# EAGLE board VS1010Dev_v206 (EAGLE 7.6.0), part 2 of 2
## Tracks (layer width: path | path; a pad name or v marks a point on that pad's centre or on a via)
3V3  (via drill 0.5)
  Top 0.2: R7.1 v96.1,27.6
  Top 0.305: C31.1 93.2,25.5 92.35,26.35 90.44,26.35 | C31.1 93.25,25.65 94.95,27.35 R7.1 | C31.1 R8.1 93.25,23.25 93.2,23.2 | CN3.4 90.35,26.35 v90.4,26.3
  Top 0.61: C37.1 29.1,20.8 29.05,20.75 U5.5 | 90.44,26.35 90.44,26.34 v90.4,26.3
  Top 1.016: C37.1 30.45,20.75 v30.5,20.8
  PWR 0.607: v96.1,27.6 96.1,34.72 JP15.7
  PWR 0.61: v30.5,20.8 37.6,20.8 39.4,22.6 40.7,22.6 42.4,20.9 42.4,15.8 43.5,14.7 47.1,14.7 50.8,18.4 50.8,19.3 52.6,21.1 60.6,21.1 61.7,22.2 81.6,22.2 85.7,26.3 v90.4,26.3
4V5  (via drill 0.5, 0.6)
  Top 0.203: U30.5 61.35,44.15 60.5,45 59.7,45 59,45.7 59,45.85 C61.2
  Top 0.25: U7.3 38.1,47.2 38.5,47.6 | 38.75,47.65 C19.1 38.5,47.6 | v39.6,48.5 39.4,48.5 38.5,47.6 | C39.1 34,51.3 34.2,51.1 U7.9 | v29.7,48.5 30.55,47.65 C17.1 30.8,47.6 31.2,47.2 U7.13 | J1.3 v30,41.2
  Top 0.305: 30.5,30.8 v32,30.8 v32,31.9 | v32,31.9 v32,33 | 30.5,30.9 30.8,30.9 31.8,31.9 v32,31.9 | J2.3 v39.2,41.2
  Top 0.406: C39.1 34.15,51.35 34.4,51.6 34.7,51.6 | 34.7,51.6 35.5,51.6 35.6,51.5 v35.6,51.4 v35.6,52.5 | 34.7,51.6 34.7,51.7 35.5,52.5 35.5,52.1 35.3,51.9 35.3,51.4 34.7,51.4
  Top 0.5: U8.6 30.14,31.16 30.5,30.8
  Top 0.6: 30.5,32.7 R21.2 30.5,30.9 C47.2 30.5,30.8
  Top 0.61: C61.2 C59.2 56.25,46.15 v56,45.9
  PWR 0.61: v39.6,48.5 39.6,48.6 39.7,48.5 46.8,48.5 48.2,47.1 48.2,46.1 49.8,44.5 54.6,44.5 v56,45.9
  pour PWR: 29.3,30.2 32.7,30.2 32.7,40.3 39.7,40.3 39.7,53.1 29.3,53.1
14
  Top 0.2: 52,24.2 52.9,23.3 54.4,23.3 56.2,21.5 57.2,21.5 59.3,19.4 59.3,13.1 60.5,11.9 63.3,11.9 64.5,10.7 64.5,2.4 64.9,2 79.6,2 80.3,2.7 80.3,10.6 85.05,15.35 85.05,15.45 R53.2 85.15,15.45 85.1,15.4
  Top 0.203: U6.14 52,24.2
16
  Top 0.2: 52.8,24 53.1,23.7 54.6,23.7 56.4,21.9 57.4,21.9 59.7,19.6 59.7,13.3 60.7,12.3 63.6,12.3 65,10.9 65,2.8 65.4,2.4 79.4,2.4 79.9,2.9 79.9,10.9 83.9,14.9 83.9,18.1 84.1,18.3 85.1,18.3 85.2,18.4 R52.2
  Top 0.203: U6.16 52.8,24
AGND  (via drill 0.5)
  Top 0.2: v34.6,40.3 v34.6,41.4 | TV4.2 25.35,45.55 25.2,45.4 25.2,40.9 25.3,40.8 | 25.3,40.8 C30.2 | 25.3,40.8 24.7,40.2 22.9,40.2 22.3,40.8 22.3,41.6 22.25,41.65 | 22.2,41.7 22.25,41.65 | 22.25,41.65 C29.2 | JMP5.1 65.05,37.4 U30.16
  Top 0.203: v61.9,44.5 62,44.4 U30.4 62,42 62.4,41.6 65.95,41.6 C10.2 67.7,41.35 JMP4.1 | C62.2 C60.2 | 56.1,41.15 C63.2
  Top 0.23: U6.58 44,30
  Top 0.25: 34,42.6 C27.2 | U7.18 34.7,43.3 34,42.6 | U7.18 34.7,43.2 35.3,42.6 C24.2 35.25,42.45 34.6,41.8 | 34,42.6 34,42.4 34.6,41.8 | v34.6,41.4 34.6,41.8 | 34.7,47.7 34,47.7 | 34,47.7 U7.12 32,47.7 | 34.7,47.7 U7.4 37.4,47.7 | U7.18 34.7,47.7 | 34,47.7 v34.1,47.8 | v34.1,47.8 v35.3,47.8 | v34.1,47.8 v34.1,46.7 35.2,46.6 v35.2,46.7 | v31.2,45.7 31.25,45.85 | 44,30 41.6,32.4 41.6,32.6 41.5,32.7 41.45,32.7 C21.2 41.15,33.05 40.2,34 38.4,34 v38.1,33.7
  Top 0.254: v41.2,55.6 41.2,51.8 42,51 | 39.85,45.85 41,47 41,50 42,51 | 42,51 42.02,50.98 | JP2.1 46.77,57.63 47.8,56.6 47.8,55.1 46.4,53.7 | 46.4,53.7 46.35,53.75 R18.2 | C33.2 47.35,50.35 46.7,51 45.3,51 45.32,50.98 | C32.1 49.3,50.4 49.25,50.35 C33.2 | 46.4,53.7 46.4,53.6 47.4,52.6 C33.2 | C33.2 47.4,50.3 | U8.8 27.65,33.75 27.7,33.8 27.35,34.15 R20.1
  Top 0.305: 16.7,40.1 v18.7,40.1 | 38.2,26.6 37.8,26.6 35.7,24.5 35,24.5 34.8,24.3 JP6.5 | C17.2 31.85,49.35 v31.9,49.3 | C19.2 37.45,49.35 v37.4,49.3 | C41.2 34,55.6 v34,54.45 C39.2 34,53.1 34.3,53.1 34.9,53.7 v35.4,53.7 | v28.5,35.8 R20.1 27.35,37.05 v27.3,37.1 | C47.1 31.95,29.05 v32,29.1 | C47.1 v30.5,27.6 | C47.1 30.55,29.05 v31.9,27.7
  Top 0.406: C41.2 34.7,55.6 | 34.7,55.6 34.8,55.6 | 34.8,55.6 C43.2 | 34.7,55.6 34.7,55.7 34.4,56 | 34.8,55.6 v34.8,56.8 | C40.2 v28.2,55.6 | v41.2,55.6 C42.2 | 22.25,46.45 22.3,46.4 | 22.25,46.45 TV3.2 | 20,46.5 v21.1,46.5 | 20,46.5 TV2.2 19.9,46.5 | v21.1,46.5 22.2,46.5 | 22.2,46.5 22.25,46.45 | v7.6,47.9 TV6.2 6.75,45.35 6.8,45.3 6.75,45.25 R40.2 v7.6,44.3 R49.2 | v7.6,47.9 TV5.2 8.5,46.8 8.5,45.2 | 8.5,45.2 7.1,45.2 6.7,44.8 6.7,43.6 6.75,43.55 C55.2 6.75,43.25 v7.6,42.4 8.5,43.3 8.5,43.5 | v7.6,47.9 v7.6,46 | v7.6,46 7.5,46.3 7.1,46.7 | v7.6,46 8.2,46.7 7.9,46.7 7.8,46.8 7.8,47 7.4,47 7.4,46.7 | v21.1,46.5 v21.1,47.6 | 20,46.5 v21.1,47.6 | v21.1,47.6 22.2,46.5 | C56.2 8.4,43.5 8.5,43.6 8.5,45.2 | C29.2 22.3,41.6 22.2,41.7 C28.2 19.95,40.95 19.1,40.1 v18.7,40.1 Q1.E | Q1.E 16.7,40.1 | Q1.E 16.75,39.95 17.55,39.15 R38.2 | J1.1 31.15,45.75 v31.2,45.7 | C32.1 51.95,50.55 v52.7,49.8 | C61.1 58.7,48.7 v57.8,49.6 57.2,49 C59.1 | JMP5.1 65.95,38.05 v66.9,37.1 | C63.2 54.3,41.1 v54,40.8 54,42.1 54.65,42.75 C60.2
  Top 0.61: C7.2 39.85,26.35 39.8,26.3 39.85,26.25 C6.2 38.6,26.2 38.2,26.6 C51.2 | C5.2 43.75,23.45 44,23.7 v44.2,24.3
  Top 1.016: C52.2 v19.2,27.1 v18,27.1 v20.4,27.1
  GND 0.2: v44.2,24.3 43.1,24.3 41.4,26
  other vias: 37.9,45.8 10.2,54 1.5,50.1 16.1,51.1 14.8,57.1 27.7,48.7 28.4,51.7 40.2,53.9 44.7,52.4 49.9,53.9 50.5,58.2 62.6,52.4 56.2,54.8 25.5,30.6 23.6,30.6 24.5,32.3 21.1,35.5 38.5,37.1 41,41.7 44.2,45.6
  pour GND (isolate 0.305): 0.1,59.9 67.3,59.9 67.4,36.8 67.2,36.6 66.4,36.6 65,38.1 49.5,38.3 49.5,28 41.6,28 41.6,25.8 35.4,25.8 35.4,24 32.5,24 32.5,26.2 11.6,26.2 11.6,41.6 0.1,41.6
  pour Top (isolate 0.254, rank 2): 0.1,41.5 11.7,41.5 11.7,26.3 32.5,26.3 32.5,22.1 49.6,22.1 49.6,38 67.3,38 67.3,59.9 0.1,59.9
  pour Bottom (isolate 0.305): 0.2,41.7 11.7,41.7 11.7,26.2 32.6,26.2 32.6,22.2 49.5,22.2 49.5,38.1 67.2,38.1 67.2,59.8 0.2,59.8
AVDD  (via drill 0.5)
  Top 0.2: 45.45,23.45 C5.1 | R33.1 18.85,19.35 18.6,19.6 18.6,21.9 18.9,22.2 v19.5,22.2 | R32.1 20.85,14.65 v20.8,14.7 | 45.29,48.61 45.27,48.61 MIC1.6
  Top 0.23: U6.63 43.6,28 v43.1,27.5 | U6.1 46.8,23.7 | U6.64 43.2,27.6
  Top 0.25: 46.8,23.7 46.2,23.1 C5.1 | 41.6,27.8 41.8,28 | C6.1 41.4,26.2 | 41.7,28 41.7,27.8 41.6,27.8 | C7.1 41.6,27.8
  Top 0.3: 43.2,27.6 v43.1,27.5 | 41.9,26.1 41.65,26.1 C6.1
  Top 0.406: 47.4,48.6 C33.1 | 47.4,48.6 47.55,48.75 C32.2 51.05,48.75 v51.1,48.8 51.2,48.7 51.1,48.6 51.1,47.9 50.6,47.4 46.3,47.4 45.8,46.9 v45.8,46.5 45.9,46.5 | 45.29,48.61 45.3,48.6 47.4,48.6
  Top 0.61: v45.5,24.7 45.45,23.45 | C51.1 38.2,28.5 37.8,28.9 v37.8,29.8 v38.9,29.8 38.9,29.4 | 38.9,29.4 38.6,29.1 38.5,29.1 38.3,29.3 38.3,29 38.2,28.9 | C6.1 41.55,26.25 41.5,26.3 41.55,26.35 C7.1 41.55,27.85 41.5,27.9 41.5,28.8 41.1,29.2 39.1,29.2 38.9,29.4 | v19.5,22.2 19.4,22.2 | 41.9,26.1 42,26.1 43.1,27.2 v43.1,27.5
  PWR 0.406: v45.8,46.5 46.2,46.1 46.2,43.7 46,43.5 46,41.7 46.6,41.1 46.6,40.6 46,40 44.5,40 42.6,38.1 42.6,33.5 v38.9,29.8 | JP1.18 81.6,38.2 | JP1.18 | JP1.18 81.5,38.2 80.2,39.5 73.2,39.5 63.9,48.8 v51.1,48.8
  PWR 0.61: v37.8,29.8 37.8,28.9 35.76,26.86 JP6.4 33.66,26.86 32.4,25.6 28.7,25.6 25.3,22.2 v19.5,22.2 | v45.5,24.7 45.45,24.95 45.5,25 45.5,25.8 43.9,27.4 43.2,27.4 v43.1,27.5 | v37.8,29.8 37.9,29.7 | v37.8,29.8 v38.9,29.8
  Bottom 0.2: v20.8,14.7 19.8,14.7 18.6,15.9 18.6,21.9 18.9,22.2 v19.5,22.2
  Bottom 0.61: 19.4,22.2 v19.5,22.2
CLK  (via drill 0.5)
  Top 0.2: 59.1,31.6 60.8,29.9 60.8,28.6 61.4,28 65.3,28 66.6,29.3 68.5,29.3 69.5,28.3 v70.7,28.3 | CN3.5 87.45,25.25 87.5,25.2
  Top 0.203: U6.32 59.1,31.6
  Top 0.406: v89,25.1 89,25.2 87.5,25.2
  Bottom 0.2: v89,25.1 89,15 86.8,12.8 72.8,12.8 72.1,13.5 72.1,17.9 70.7,19.3 v70.7,28.3
CMD  (via drill 0.5)
  Top 0.2: 58.9,31.2 60.4,29.7 60.4,28.4 61.2,27.6 65.5,27.6 66.8,28.9 68.3,28.9 70,27.2 v72,27.2 | v89,27.5 87.6,27.5 87.5,27.4
  Top 0.203: U6.31 58.9,31.2
  Top 0.305: 87.5,27.4 87.45,27.4 CN3.3
  Top 0.406: R7.2 89.1,27.6 v89,27.5
  Bottom 0.2: v89,27.5 88.1,26.6 88.1,14.8 86.5,13.2 73,13.2 72.5,13.7 72.5,18.1 71.1,19.5 71.1,26.3 v72,27.2
CVDD  (via drill 0.5)
  Top 0.2: 50,35.9 50.8,36.7 C8.1 50.85,36.75 | 47.6,22.9 46.9,22.2 46.9,21.1 47.6,20.4 48,20.4 48.3,20.1 C9.1
  Top 0.203: v45,17 40.1,17 39.9,17.2 38.2,17.2 37.2,18.2 37.2,19.5 | 37.2,19.5 37.2,19.8 36.8,20.2 | D6.ANODE 37.14,19.56 37.2,19.5 | U6.3 47.6,22.9 | U6.43 50,35.9
  Top 0.406: v51.9,37.8 50.85,36.75
  Top 0.5: R3.1 70.35,50.35 70.8,50.1 v70.8,49.1
  Top 0.61: v45,17 v45,18.1 44.9,18.2 45.95,19.25 C49.1 46.5,19.3 46.55,19.35 C9.1
  PWR 0.406: JP1.11 68.87,45.83 68.15,46.55 64.3,50.4 62.8,50.4 61.7,51.5 59.7,51.5 58.9,50.7 51.4,50.7 49.9,49.2 49.9,48.2 52.4,45.7 54.4,45.7 55.5,46.8 57.6,46.8 58.3,46.1 58.3,44.2 55.6,41.5 55.6,40.7 52.7,37.8 v51.9,37.8
  PWR 0.5: v70.8,49.1 70.7,49.1 68.15,46.55
  PWR 0.61: v45,18.1 45,20.3 48.9,24.2 50.6,24.2 53.8,27.4 53.8,36 52,37.8 v51.9,37.8
DAT0
  Top 0.2: 87.4,23 87.45,23.05 | 87.4,23 89.3,23 90.1,22.2 93.9,22.2 94.95,23.25 R8.2 94.95,23.35 95,23.3 95,22.2 92.5,19.7 87.4,19.7 85.8,21.3 85.8,29.8 82.1,33.5 78.1,33.5 76.5,35.1 74.5,35.1 72,37.6 | 55.9,37.8 55.7,37.6 55.7,37.1 55.3,36.7 54.5,36.7 52,34.2 | CN3.7 87.4,23
  Top 0.203: U6.38 52,34.2 | 55.9,37.8 57.1,39 66.4,39 67.7,37.7 71.9,37.7 72,37.6
DAT1
  Top 0.2: 87.3,21.9 87.4,22 87.45,21.95 87.4,21.9 87.2,22.1 86.9,22.1 86.2,22.8 86.2,30.9 85.99,31.11 arc90 85.58,31.11 arc-90 85.17,31.11 85.15,31.13 arc-90 85.15,31.54 85.56,31.95 arc90 85.56,32.37 85.53,32.39 arc90 85.12,32.39 84.71,31.98 arc-90 84.3,31.98 84.27,32.01 arc-90 84.27,32.42 84.68,32.83 arc90 84.68,33.24 84.66,33.26 arc90 84.25,33.26 83.84,32.85 arc-90 83.43,32.85 83.4,32.88 arc-90 83.4,33.29 arc90 83.4,33.7 83.2,33.9 78.3,33.9 76.7,35.5 74.7,35.5 72.2,38 | 55,39 54.3,39 53.9,38.6 53.9,37.3 51.2,34.6
  Top 0.203: U6.40 51.2,34.6 | 55,39 56.5,39 56.9,39.4 66.6,39.4 67.9,38.1 72.1,38.1 72.2,38
  Top 0.305: 87.4,22 CN3.8
DAT2
  Top 0.2: 55.2,39.4 54.1,39.4 53.5,38.8 53.5,37.5 50.8,34.8 | 72.4,38.4 74.9,35.9 76.9,35.9 78.5,34.3 84.1,34.3 84.35,34.05 arc90 84.76,34.05 85.7,34.99 arc-90 86.11,34.99 86.18,34.92 arc-90 86.18,34.51 85.24,33.57 arc90 85.24,33.16 85.31,33.09 arc90 85.72,33.09 86.66,34.03 arc-90 87.07,34.03 87.14,33.96 arc-90 87.14,33.55 86.2,32.61 arc90 86.2,32.2 86.27,32.13 arc90 86.68,32.13 87.62,33.07 arc-90 88.03,33.07 88.09,33.01 arc-90 88.09,32.59 87.16,31.66 arc90 87.16,31.24 87.5,30.9 87.5,29.75 CN3.1
  Top 0.203: U6.41 50.8,34.8 | 55.2,39.4 56.3,39.4 56.7,39.8 66.8,39.8 68.1,38.5 72.3,38.5 72.4,38.4
DAT3  (via drill 0.5)
  Top 0.2: 58.7,30.8 60,29.5 60,28.2 60.8,27.4 60.8,25.95 61.28,25.47 65.98,25.47 v66.05,25.4 66.1,25.4 66.05,25.45 | 87.45,28.55 87.4,28.6 v89,28.6
  Top 0.203: U6.30 58.7,30.8
  Top 0.305: CN3.2 87.4,28.6
  Bottom 0.2: v89,28.6 91,28.6 92.5,27.1 92.5,22.6 90.3,20.4 90.3,15.7 87,12.4 72.5,12.4 71.7,13.2 71.7,17.7 70.3,19.1 70.3,20.3 66.05,24.55 v66.05,25.4
GBUF
  Top 0.2: U6.61 43.2,28.8
  Top 0.25: U7.20 35.7,44.7 36.6,43.8 37.6,43.8 37.9,43.5 37.9,39.1 36.5,37.7 35,37.7 | U7.16 33.7,44.7 32.8,43.8 31.6,43.8 31.3,43.5 31.3,39.1 32.7,37.7 34.4,37.7 | 34.4,37.7 35,37.7 | 34.7,37.4 34.4,37.7 | 34.7,37.4 35,37.7 | 34.7,37.4 34.7,36.1 34.3,35.7 33.1,35.7 32.9,35.7 32.8,35.6 32.6,35.4 32.6,33.7 34.36,31.94 JP6.2 34.86,31.94 34.9,31.9 36.6,31.9 37.4,31.1 40.9,31.1 43.2,28.8
  Top 0.406: R6.1 26.35,44.25 26.4,44.3 26.65,44.05 | 27,43.7 28.6,42.1 28.6,39.8 32.8,35.6 32.8,35.4 | 27,43.7 26.65,44.05 | 26.65,44.05 27,44.4 | 27,44.4 27.7,45.1 27.7,46.7 27.2,47.2 26.2,47.2 TV4.1 26.2,55 26.8,55.6 CN6.5 | 27,44.4 27,44.5 26.7,44.5 | 27,43.7 27,44.4 | 32.8,35.4 33.1,35.7 32.8,35.7 | 32.8,35.4 32.6,35.4 32.6,35.6
GND  (via drill 0.3, 0.5)  (1 unrouted)
  Top 0.2: C50.2 49.95,17.55 49.9,17.6 C3.2 48.35,17.65 48.3,17.6 C9.2 46.65,17.65 46.5,17.5 C49.2 v46.5,16.1 | C11.2 44.4,19 v43.6,18.2 42.6,19.2 C48.2 44.25,19.65 44.3,19.7 | U2.29 75.05,24.95 v74.7,24.6 | JP11.8 64.49,23.99 64.5,24 66.4,24 66.85,24.45 U2.9 68.95,24.45 v69,24.4 | C38.2 v70.6,35.5 | C2.2 73.85,33.75 73.95,33.85 C1.2 75.65,33.85 77.1,32.4 v77.1,31.9 | U2.4 68.95,26.95 v69,27 | U2.47 69.65,29.25 69.8,29.1 71.6,29.1 71.8,28.9 v71.8,28.3 | R22.1 12.6,10.6 12.1,10.1 12.1,9.8 11.8,9.5 11.8,9.2 10.8,8.2 v10.8,6.8 | C12.1 47.1,46.3 | 52.1,46.2 C13.1 | TV1.2 v96.8,46.1 | C18.2 68.65,52.35 v69.3,53
  Top 0.203: U6.22 53.54,27.6 53.41,27.74 51.91,27.74 | 51.91,27.74 51.5,28.1 | 48,27.3 48.1,27.3 U6.P$1 | 51.95,27.25 51.95,27.65 51.91,27.74
  Top 0.25: 38.74,23.34 C14.2 | U2.13 69.15,20.15 v69.2,20.1 69.8,19.5 70.9,19.5 70.96,19.44 | 70.96,19.44 71,19.4 | C57.2 70.96,19.44
  Top 0.254: 47.1,46.3 48.6,46.3 48.9,46.6 49.5,46.6 | 52.1,46.2 50.5,46.2 50.1,46.6 49.5,46.6 | 49.5,46.6 v49.5,46.5
  Top 0.3: XT1.4 v47,43
  Top 0.305: C35.1 83.85,30.35 v84.8,29.4 | C34.1 84.65,22.85 v84.7,22.9 | C31.2 95,25.5 v96,24.5 | CN3.6 90.55,24.15 v90.6,24.2 | CN3.9 v91.8,20.8
  Top 0.4: C4.2 48.3,39.3 v48.3,39.9 | C8.2 50.8,40 v50.7,40.1
  Top 0.406: X1.5 6.01,15.12 v6.5,15 v5.2,15 | v5.2,15 v7.8,15 6.9,15.7 | v5.2,15 5,15.5 5.2,15.7 | BATT2.NEG v53.3,5.9 | C45.2 64.15,19.65 64.5,20 v64.5,21 | C15.1 v40.1,40 | C16.1 v41.7,40
  Top 0.5: XT1.2 v50.7,40.1
  Top 0.6: RESET.A 68.9,58.5 v70.4,57 71.9,58.5 RESET.A1
  Top 0.61: 38.74,23.34 38.54,23.34 v37.6,22.4 | 25.6,23.2 25.6,23.1 24.95,22.45 C36.2 22.1,22.9 v22.8,23.6 | 25.6,23.2 U5.2 25.6,25.7 | C37.2 26.35,22.45 25.6,23.2 | 25.6,25.7 25.65,25.75 R12.2 25.65,27.15 v25.6,27.2 | C37.2 30.45,22.45 v30.5,22.5 | C37.2 v29.1,23.7 | 25.6,25.7 v24.3,25.7
  GND 0.2: 48.5,30.7 49.8,30.7 50,30.5 U6.P$5 51.2,29.2
  GND 0.4: v48.3,39.9 50.5,39.9 v50.7,40.1
  GND 0.5: v47,43 49.7,43 50.7,42 v50.7,40.1 50.7,31.5 50.6,31.4 49.2,31.4 48.5,30.7 48.5,31.4 41.8,38.1 41.8,39.9 v41.7,40 v40.1,40
  GND 0.61: v37.6,22.4 37.6,21.1
  Bottom 0.152: U$37.C3 U$37.B3 78.5,17.9 78,17.4 76,17.4 75.6,17 v75.6,16.1
  Bottom 0.3: v49.5,46.5 49.5,45.4 47.1,43 v47,43 46.5,42.5 44.4,42.5 41.9,40 v41.7,40 v40.1,40
  other vias: 98,10.2 14.6,1.4 8.2,24.6 6.6,7.2 36,3.3 2.2,16.7 98.4,16.3 23.5,6.8 24.6,18.5 16.2,14.8 12.6,24.4 29.5,18.6 35.7,18.6 9.5,21.3 19.9,24.3 87.6,47.4 88.3,55.7 98.8,54.9 93.9,33.3 83.2,10.2 67.7,43.5 70.9,48 65.9,30 52.8,10.6 35.2,12.3 71.2,10.8 31.8,3.3 40.2,4.6 56,10.6 56.7,12.8 89.2,31.3
  pour GND (isolate 0.305): 0.1,41.1 11.1,41.1 11.1,25.7 32,25.7 32,23.5 35.9,23.5 35.9,25.3 42.1,25.3 42.1,27.5 46.8,27.5 46.8,31.9 50,31.9 50,37.6 59.8,37.5 60.3,38.6 63,38.6 63.6,37.5 64.6,37.5 65.9,36.2 67.8,36.2 67.8,59.9 99.9,59.9 99.9,0.1 94.2,0.1 94.2,2.4 88,2.4 88,0.1 0.1,0.1
  pour Top (isolate 0.254): 0.1,40.8 11.1,40.8 11.1,25.7 31.9,25.7 31.9,21.5 50.2,21.5 50.2,37.4 67.9,37.4 67.9,59.9 99.9,59.9 99.9,0.1 94.2,0.1 94.2,2.4 88,2.4 88,0.1 0.1,0.1
  pour Bottom (isolate 0.305): 0.2,41.1 11.1,41.1 11.1,25.6 32,25.6 32,21.6 50.1,21.6 50.1,37.5 67.8,37.5 67.8,59.8 99.8,59.8 99.8,0.2 94.2,0.2 94.2,2.3 88,2.4 88,0.2 0.2,0.2
GP27  (via drill 0.5)
  Top 0.2: 54.8,26.8 55.1,26.5 55.1,25.7 55.2,25.6 v57.7,25.6
  Top 0.203: U6.20 54.8,26.8
  Bottom 0.2: v57.7,25.6 58,25.6 58.4,25.2 58.8,25.2 61.1,22.9 65,22.9 65.6,23.5 65.6,24.5 65.2,24.9 65.2,25.7 68.5,29 68.5,30.2 68,30.7 68,32.9 68.6,33.5 84.4,33.5 88.4,37.5 95.4,37.5 JP15.5
HPDET
  Top 0.305: R24.1 13.35,41.65 14.4,42.7 14.4,53.1 17.5,56.2 CN6.6
I2S_12M  (via drill 0.5)
  Top 0.2: JP11.1 61.91,31.61 61.9,31.6 60.7,32.8 U30.11 | 58.5,30.4 59.6,29.3 59.6,27.6 60.1,27.1 v60.05,27.05
  Top 0.203: U6.29 58.5,30.4
  Bottom 0.2: 60.1,27 v60.05,27.05 60.15,27.05 60.2,27 60.6,27 60.8,26.8 60.8,25.9 61.23,25.47 62.47,25.47 63,26 63,30.6 61.99,31.61 JP11.1
I2S_BCK  (via drill 0.5)
  Top 0.2: 54.3,33.2 v55,33.9
  Top 0.203: U6.35 54.3,33.2 | U30.12 61.35,36.15 61.5,36 62.4,36 63.4,35 63.4,32.68 JP11.2
  Bottom 0.2: 64.49,31.61 64.5,31.6 | 64.49,31.61 JP11.2 | 64.49,31.61 63.4,32.7 56.6,32.7 55.4,33.9 v55,33.9
I2S_DI
  Top 0.2: JP11.3 61.93,29.37 59.3,32 57.9,32
  Top 0.203: U6.33 55.3,32 55.6,32 57.9,32
  PWR 0.3: JP16.P$1 63.2,33.5 63.2,29.9 62.37,29.07 JP11.3
I2S_DO  (via drill 0.5)
  Top 0.2: 54.9,32.4 v55.3,32.8
  Top 0.203: U6.34 54.9,32.4
  Bottom 0.2: 61.97,26.53 62,26.5 | 61.97,26.53 JP11.5 | 61.97,26.53 59.6,28.9 59.6,29.3 58.5,30.4 57,30.4 55.3,32.1 v55.3,32.8
I2S_FRM
  Top 0.2: JP11.4 64.5,29.1 63.2,30.4 61.5,30.4 59.5,32.4 58.2,32.4 56.7,33.9 56.7,34.7 56.65,34.75 56.65,35.2 | 56.65,35.2 56.65,35.65 56.4,35.9 55,35.9 52.8,33.7 | U30.10 60.05,38.45 59.9,38.6 58.9,38.6 58.7,38.4 58.7,36.4 57.9,35.6 57.05,35.6 56.65,35.2
  Top 0.203: U6.36 52.8,33.7
IOVDD  (via drill 0.4, 0.5, 0.6)
  Top 0.2: 47.95,36.85 48.8,36 | C4.1 47.85,36.85 47.8,36.8 | 48,22.5 47.4,21.9 47.4,21.2 47.8,20.8 49.3,20.8 49.9,20.2 C3.1 | v52.8,42.8 52.85,42.75 | v69.4,32.1 69.45,32.05 | R2.1 43.25,14.85 43.7,14.4 49,14.4 v49.9,15.3 | 54.3,12.7 54.3,14.6 54.66,14.96 U4.3 | 54.3,12.7 53.5,11.9 v49.9,11.9 | R58.1 66.4,33.75 | R54.1 2.65,8.15 3,7.8 v3,5.4 | R62.2 14.1,13.1 14.4,13.4 20,13.4 20.3,13.1 R59.2 19.45,12.35 18.9,11.8 18.9,5.5 v19,5.4 | R30.2 37.2,10.6 36.3,9.7 36.3,8 v36.4,7.9 | R31.2 28.85,10.65 27.7,9.5 v27.7,7.4 | U4.7 U4.8 62.81,19.14 C45.1 | 54.3,12.7 55,12 57.2,12 59.3,9.9 60,9.9 v60.4,10.3
  Top 0.203: U6.4 48,22.5 | U6.46 48.8,36 | 62.65,36.45 64.4,34.7 65.65,34.7 JMP5.3 65.7,33.5 v65.9,33.3 66.35,33.75 66.4,33.75 | U30.13 62,36.5 62.1,36.4 62.6,36.4 62.65,36.45 | U30.14 62.65,36.45 | JMP4.3 70.45,39.65 v70.7,39.4 | U30.6 60.7,44.1 60.3,44.5 57.75,44.5 C62.1
  Top 0.25: C38.1 70.55,32.05 70.5,32 71.15,31.35 U2.44 | U2.38 74.15,31.75 73.85,32.05 | C57.1 72.55,19.55 71.65,20.45 U2.18 | U2.40 73.15,31.25 73.5,31.6 73.5,31.75 C2.1
  Top 0.406: C3.1 49.9,19.3 49.95,19.25 C50.1 51.5,19.2 51.7,19 52.1,19 53,18.1 v53,17.9 | v46.5,37.8 46.8,37.8 47.5,37.1 47.7,37.1 47.95,36.85 C4.1 | D2.C 95.7,17.7 95.45,17.45 R46.1 | v69.4,32.1 69.5,32.1 69.55,32.05 C38.1 | 75.45,32.15 75.4,32.2 C1.1 75.4,32.1 73.9,32.1 73.85,32.05 C2.1 | 62.31,19.31 62.5,19.5 C45.1 v61.3,19.5 | R29.1 50.1,15.5 v49.9,15.3
  Top 0.61: C57.1 73.66,19.44 v73.7,19.4 | D1.C 67.7,17.8 67.9,17.6 69.5,17.6 69.6,17.5 R43.1 70.75,17.55 v70.8,17.5 70.85,17.55 R42.1 75.45,17.55 D12.C | R46.1 93.6,17.5 v91.5,17.5 91.45,17.45 R47.1 89.55,17.45 89.3,17.7 D3.C | R9.1 94.95,29.75 94.9,29.8 v94.9,31.4 | 75.4,32.1 75.4,31 v75.6,30.8 | v83.5,43.6 R34.2 | v73.6,51.8 R35.2 | C62.1 C60.1 54.45,44.45 | 54.45,44.45 v52.8,42.8 | v53.8,46.6 53.8,45.1 54.45,44.45
  PWR 0.2: 28,7.1 v27.7,7.4 | 83.6,33.7 83.5,33.7 83.4,33.8 82.7,33.8 | 83.5,33.8 83.5,34.5 | v60.4,10.3 64.59,10.3 JP5.2
  PWR 0.254: 81.7,58.4 81.6,58.4 80.4,57.2 78.2,57.2 77.3,56.3 77.3,55.4 v73.6,51.8
  PWR 0.406: 64.6,26.5 66.5,26.5 70.2,30.2 | 70.75,30.75 70.3,30.3 | 70.3,30.3 70.2,30.2 | 70.3,31.2 70.3,30.3 | 70.2,30.2 71.2,30.2
  PWR 0.6: v70.7,39.4 66.1,39.4 65.9,39.2
  PWR 0.61: v3,5.4 v19,5.4 26.3,5.4 28,7.1 28.8,7.9 v36.4,7.9 40.9,7.9 45.6,3.2 48.1,3.2 49.9,5 v49.9,11.9 v49.9,15.3 52.4,15.3 | v75.6,30.8 75.7,30.7 75.6,30.7 | v52.8,42.8 51.5,42.8 49.5,40.8 49.5,39.3 48,37.8 v46.5,37.8 | 75.6,30.7 75.6,33.3 76.1,33.8 82.6,33.8 83.05,34.25 | 83.05,34.25 83.5,34.7 v83.5,43.6 83.5,56.6 81.7,58.4 JP1.2 | 83.05,34.25 83.5,33.8 83.6,33.7 88.6,33.7 90.9,31.4 v94.9,31.4 94.4,30.9 94.4,18.9 93,17.5 v91.5,17.5 90.8,18.2 v83,18.2 74.9,18.2 v73.7,19.4 71.8,17.5 v70.8,17.5 67.8,17.5 65.9,19.4 61.4,19.4 v61.3,19.5 57.1,15.3 53.6,15.3 | 64.6,26.5 64.57,26.53 JP11.6 | 53.6,15.3 53,15.3 | v53,17.9 53,15.9 | 53,15.9 53,15.3 | 53,15.3 52.4,15.3 | 52.4,15.3 53,15.9 | 53,15.9 53.6,15.3 | 75.6,30.7 75.5,30.7 74.9,30.1 71.4,30.1 70.75,30.75 70.3,31.2 v69.4,32.1 67.6,32.1 66.2,33.5 v65.9,33.3 65.9,39.2 65.9,42.2 60.4,47.7 54.9,47.7 v53.8,46.6
  Bottom 0.152: U$37.B4 78.7,16.6 78.2,16.1 78.2,15.2 77.4,14.4 74.9,14.4 74.2,15.1 74.2,18.9 v73.7,19.4
  Bottom 0.2: U$37.E2 82.3,18.9 v83,18.2
KB1
  Top 0.2: CN2.8 87.2,12.2 86.5,12.9 86.5,16.2 86,16.7 85.2,16.7 R52.1
KB2
  Top 0.2: CN2.2 89.3,9.1 88.4,10 86.5,10 85.2,11.3 85.2,13.6 85.1,13.7 85.15,13.75 R53.1
KCLK
  Top 0.2: 51.2,23.8 52.5,22.5 54,22.5 55.8,20.7 56.8,20.7 58.5,19 58.5,12.7 60.1,11.1 62.5,11.1 63.5,10.1 63.5,1.8 64.2,1.1 80,1.1 81.2,2.3 81.2,7 82.2,8 85.4,8 86.3,7.1 94.4,7.1 95.2,7.9 95.2,10.1 95.6,10.5 D2.A
  Top 0.203: U6.12 51.2,23.8
  Top 0.406: R46.2 93.6,14.5 94,14.1 R45.1 95.4,14.1 D2.A
KCLK1
  Top 0.406: R45.2 92.25,11.75 92.8,11.2 CN2.6 94.1,11.2
KDATA
  Top 0.2: 51.6,24 52.7,22.9 54.2,22.9 56,21.1 57,21.1 58.9,19.2 58.9,12.9 60.3,11.5 63,11.5 64,10.5 64,2.2 64.6,1.6 79.9,1.6 80.8,2.5 80.8,7.2 82,8.4 85.6,8.4 86.5,7.5 90.2,7.5 90.6,7.9 90.6,10.9 89.3,12.2 89.3,14.05 R48.2
  Top 0.203: U6.13 51.6,24
  Top 0.406: D3.A 87.7,13.9 87.9,14.1 R48.2 89.3,14.1 89.6,14.4 R47.2
KDATA1
  Top 0.406: CN2.1 91.9,10.9 91,11.8 91,14.1 R48.1
L+
  Top 0.406: L4.2 38.7,54.4 38.4,54.7 38.4,55.4 38.3,55.5 38.35,55.55 C42.1 38.35,56.75 38.9,57.3 38.9,58.2 39,58.3 38.97,58.33 JPL.1
LEFT  (via drill 0.5)
  Top 0.23: U6.62 42.9,28.4
  Top 0.25: R14.2 36.55,39.65 v35.5,38.6 | JP6.3 35.3,29.4 36.5,30.6 40.7,30.6 42.9,28.4
  Top 0.406: R51.1 1.95,43.15 v2.8,42.3 | 19.9,43.2 19.95,43.25 R4.1 R16.1 v21.1,44.9
  Bottom 0.406: JP6.3 35.4,29.4 37.2,31.2 37.2,36.9 v35.5,38.6 35.1,38.6 33.8,39.9 26.1,39.9 v21.1,44.9 15,44.9 14.1,45.8 10.7,45.8 8.3,43.4 3.9,43.4 v2.8,42.3
MISO0  (via drill 0.4, 0.5)
  Top 0.2: 49.6,23 51.7,20.9 52.7,20.9 53,20.6 53,19.6 54.2,18.4 55.2,18.4 | 55.2,18.4 v55.2,18.5 | 55.2,18.4 57.6,18.4 58.1,17.9 58.1,16.8 58,16.7 | 58,16.7 57.6,16.3 55.45,16.3 U4.2 53.59,16.23 | U2.3 66.95,27.45 66.8,27.3 66.8,25 66.4,24.6 65.5,24.6 65.05,25.05 63.55,25.05 63.2,24.7 63.2,23.4 62.7,22.9 61.1,22.9 60.4,23.6 v58,23.6 | 58,16.7 58,12.3 v59.5,10.8
  Top 0.203: U6.8 49.6,23
  Top 0.406: 53.59,16.23 R29.2
  GND 0.2: v77.9,21.2 77.9,19.3 77,18.4 66.5,18.4 65.8,19.1 64,19.1 63.7,19.4 63.7,21.9 62.8,22.8 60.1,22.8 59.3,23.6 v58,23.6
  PWR 0.2: v59.5,10.8 59.6,10.8 59.9,11.1 65.9,11.1 68.7,8.3 68.7,6.19 JP5.3
  Bottom 0.152: U$37.D2 80.4,18.9 79.9,19.4 79.4,19.4 79.2,19.6 79.2,20.2 78.2,21.2 v77.9,21.2
  Bottom 0.2: v55.2,18.5 55.2,20.8 v58,23.6
MISO1  (via drill 0.5)
  Top 0.2: 57.2,27.9 v57.2,28 57,28 56.6,27.6 55.8,27.6 55,28.4 | v72.2,36.3 R28.1
  Top 0.203: U6.24 55,28.4
  Bottom 0.2: v57.2,28 57,28 56.6,27.6 55.8,27.6 55,28.4 55,29.3 52.6,31.7 52.6,35 53.9,36.3 57.8,36.3 59.3,37.8 73.5,37.8 73.55,37.75 | 79.09,43.29 79.1,43.3 | 79.09,43.29 JP1.13 | v72.2,36.3 72.2,36.4 73.55,37.75 | 73.55,37.75 79.09,43.29
MISO1_  (via drill 0.5)
  Top 0.2: U2.42 72.15,31.15 v72.2,31.2 R28.2
  GND 0.2: v72.2,31.2 73.7,31.2 77.6,27.3 77.6,23.7 78.9,22.4 79.9,22.4 81.7,20.6 81.7,17.3 82.1,16.9 v83,16.9
  Bottom 0.3: U$37.E4 v83,16.9
MOCLK  (via drill 0.5)
  Top 0.2: 54,24.8 54.3,24.5 55,24.5 56.8,22.7 57.8,22.7 59.7,20.8 62.2,20.8 v62.4,21 | v66,13.7 66,14.4 68.3,16.7 71.4,16.7 72.2,15.9 73.65,15.9 R42.2
  Top 0.203: U6.18 54,24.8
  Top 0.406: D12.A 75.7,14.1 75.6,14.2 R41.2 74.05,14.25 74,14.3 74.1,14.4 74.1,15.3 73.7,15.7 R42.2
  Bottom 0.2: v66,13.7 66,15.4 64.1,17.3 64.1,19.3 v62.4,21
MOCLK1
  Top 0.2: R41.1 72.3,14.2
  Top 0.406: R41.1 72.35,12.65 73.9,11.1 77.9,11.1 79.1,9.9 79.1,5.4 78.7,5 77.79,5 JP5.9
MODATA
  Top 0.2: 53.2,24.3 53.4,24.1 54.8,24.1 56.6,22.3 57.6,22.3 60.1,19.8 60.1,13.5 60.9,12.7 66.4,12.7 67.1,13.4 67.1,13.5 D1.A
  Top 0.203: U6.17 53.2,24.3
  Top 0.406: D1.A 67.6,14.1 67.7,14.2 69.2,14.2 | R43.2 69.6,15.8 69.2,15.4 69.2,14.2 | 69.2,14.2 R44.1
MODATA1
  Top 0.2: R44.2 70.95,14.15
  Top 0.406: R44.2 71,14.2 71,12.7 73.9,9.8 76.3,9.8 77.58,8.52 JP5.10
MOSI0  (via drill 0.4, 0.5)
  Top 0.2: 74.7,21.4 U2.24 74.65,20.15 | v57.5,38.2 56.2,37 55.5,36.3 54.7,36.3 52.4,34 | R59.1 20.35,10.6 21.2,10.6 21.5,10.3 B2.A1 B2.A 21.5,1.5 21.9,1.1 48.1,1.1 49,2 61.2,2 62.2,3 v62.2,9.4 | 74.65,20.15 74.65,18.75 74.3,18.4 70,18.4 69.4,19 66.8,19 66.6,18.8 66.6,15.7 64.69,13.79 64.69,13.7 v64.41,13.7 v64.4,13.7 v64.39,13.7 U4.5 | 74.65,20.15 v74.6,20.2
  Top 0.203: U6.37 52.4,34
  PWR 0.2: v64.4,13.7 64.5,13.7 65.5,12.7 66.9,12.7 69.9,9.7 72.6,9.7 73.77,8.53 73.77,6.26 75.04,4.99 JP5.7
  Bottom 0.152: U$37.D3 80.2,17.4 78.5,17.4 78.2,17.1 78.2,16.6 78,16.4 77,16.4 75.7,15.1 75,15.1 74.65,15.45 74.65,20.15 v74.6,20.2
  Bottom 0.2: v64.4,13.7 64.5,13.7 65.2,14.4 65.2,15.5 63.8,16.9 61.5,16.9 60.5,17.9 60.5,22.8 58.5,24.8 56.1,24.8 53.8,27.1 53.8,28.7 51.4,31.1 51.4,35.6 53.3,37.5 56.7,37.5 v57.5,38.2 | v62.2,9.4 62.2,10.4
  Bottom 0.25: 62.2,10.4 64.4,12.6 v64.4,13.7
MOSI1  (via drill 0.5)
  Top 0.2: 54.8,28 55.6,27.2 56.7,27.2 56.9,27 v56.9,26.9 | JP1.12 81.57,45.87 81.6,45.9 81.7,45.8 84.4,45.8 86.9,43.3 91,43.3 92.8,41.5 92.95,41.5 R26.2
  Top 0.203: U6.23 54.8,28
  Bottom 0.2: v56.9,26.9 56.9,27 56.7,27.2 55.6,27.2 54.6,28.2 54.6,29.1 52.2,31.5 52.2,35.2 53.7,36.7 57.6,36.7 59.1,38.2 72.2,38.2 78.6,44.6 80.4,44.6 81.6,45.8 JP1.12
N$1  (via drill 0.6)
  other vias: 7.2,22.5
N$2
  Bottom 0.2: 77.2,15 76.8,15 76.8,15.4
N$3
  Top 0.2: XT4.1 40.05,35.55 40.1,35.6 C15.2
  Top 0.23: U6.57 44.2,30.4
  Top 0.25: XT4.1 40.05,35.35 40.6,34.8 40.6,34.6 41.2,34 42.1,34 42.4,33.7 42.4,32.2 44.2,30.4
N$4
  Top 0.2: C16.2 41.7,37.1 42.1,36.7 42.1,35.9 42.55,35.45 XT4.2
  Top 0.23: U6.56 44.5,30.8
  Top 0.25: 42.6,35.2 42.55,35.25 XT4.2 42.55,34.95 42.5,34.9 42.5,34.5 42.9,34.1 42.9,32.4 44.5,30.8
N$5
  Bottom 0.2: 82.6,15.4 82.6,15 82.2,15
N$6
  Top 0.2: B1.B B1.B1 33.9,9.9 33.5,10.3 33.05,10.6 R60.1
N$7  (via drill 0.6)
  other vias: 4.8,22.5
N$8  (via drill 0.5)
  Top 0.2: v55.9,26.35 55.8,26.4 55,27.2 | v73.9,41.2 73,42.1 73,49.6 72.3,50.3 72.3,50.55 R3.2 72.25,53.85 72.9,54.5 | 72.9,54.5 RESET.B1 | C18.1 66.95,54.35 RESET.B 72.9,54.5
  Top 0.203: U6.21 55,27.2
  Bottom 0.2: v55.9,26.35 55.85,26.35 54.2,28 54.2,28.9 51.8,31.3 51.8,35.4 53.5,37.1 57.4,37.1 58.9,38.6 71.3,38.6 v73.9,41.2
N$9  (via drill 0.6)
  other vias: 3,22.5
N$10  (via drill 0.6)
  other vias: 7.2,12.4
N$11
  Top 0.23: U6.59 43.8,29.6
  Top 0.25: 43.8,29.6 41.3,32.1 40.1,32.1 39.45,32.75 C21.1
N$12
  Top 0.2: PWR.A PWR.A1
  Top 0.254: C44.1 R23.1 9.45,10.8 5.1,10.8 4.7,10.4 PWR.A1
N$13
  Top 0.2: C58.1 60.45,48.15 57.9,50.7 57.9,50.9 CN8.4
N$14
  Top 0.2: 44.7,33.4 44.7,33.8 43.5,35 43.5,36.4 42.8,37.1 42.8,47.8 42.2,48.4 42.07,48.53 | 42.02,48.62 42,48.6 42.07,48.53 | MIC1.4 42.07,48.53
  Top 0.23: U6.54 45.1,31.6
  Top 0.25: 45.1,31.6 44.7,32 44.7,33.4
N$15
  Top 0.305: Q1.B 14.85,40.05 14.9,40 14.85,39.95 R24.2
N$16
  Top 0.2: 47.2,23.3 46.4,22.5 46.4,22.2 45.9,21.7 44.7,21.7 44.4,21.4 C11.1
  Top 0.23: U6.2 47.2,23.3
  Top 0.61: C11.1 44.35,21.45 44.25,21.35 C48.1 40.05,21.35 39.86,21.16 JP8.1
N$17
  Top 0.406: 23.9,46.5 TV3.1 | CN6.1 23.6,46.8 23.9,46.5 | R17.2 23.8,44.9 23.9,45 23.9,46.5
N$18
  Top 0.406: C28.1 18.25,41.55 | 18.25,41.55 R4.2 | 18.25,41.55 18.2,41.5
N$19
  Top 0.406: C29.1 23.95,41.55 | 23.95,41.55 R5.2 | 23.95,41.55 23.9,41.5
N$20
  Top 0.305: R6.2 26.25,42.55 27,41.8 27,40.8 C30.1
N$21
  Top 0.254: U8.2 19.36,32.45 18.5,33.3 16.7,33.3 R63.2
  Top 1: 13.26,33.42 JP3.1 13.23,33.4 R63.2
  Top 1.016: JP3.1 13.67,32.97
N$22
  Top 0.406: R16.2 18.2,44.9 18.25,44.95 TV2.1 18.25,46.55 18.2,46.6 18.4,46.8 CN6.4
N$23
  cutout Top: 14.7,34.3 14.7,29.6 22.5,29.6 22.5,34.3
N$24
  Top 0.203: U30.1 66.15,43 C10.1
N$25
  Top 0.305: R9.2 93.2,29.7 92.4,30.5 CN3.12
N$26
  Top 0.406: R50.2 11.55,43.85 11.9,44.2 C54.1 | R50.2 11.6,43.5 | C56.1 R50.2
N$27
  Top 0.2: C46.1 62.6,49.1 61.5,50.2 CN8.1
N$28  (via drill 0.3)
  other vias: 89.6,20.8
N$31
  Top 0.2: 45.2,33.4 45.2,33.9 43.9,35.2 43.9,36.6 43.2,37.3 43.2,47.8 43.7,48.3 43.7,48.31 MIC1.5
  Top 0.23: 45.2,32.2 arc90 45.4,32 U6.53
  Top 0.25: 45.4,32 45.2,32.2 45.2,33.4
N$32
  Top 0.2: R13.1 32.65,41.35 32.2,41.8 32.2,42.6 C27.1
  Top 0.25: U7.17 34.2,44.5 32.3,42.6 C27.1
N$33
  Top 0.2: R14.1 36.65,41.35 37.1,41.8 37.1,42.4 36.9,42.6 C24.1
  Top 0.25: C24.1 36.95,42.65 35.2,44.4 U7.19
N$34
  Bottom 0.2: 76.8,20.4 76.8,20.8 77.2,20.8
N$35
  Bottom 0.2: 82.2,20.8 82.6,20.8 82.6,20.4
N$36
  Top 0.2: X1.4 9.25,16.7 R11.1
N$37
  cutout Bottom: 77,15.2 82.4,15.2 82.4,20.6 77,20.6
N$38  (via drill 0.6)
  other vias: 4.9,12.4
N$39  (via drill 0.5)
  Top 0.2: v48.2,21.6 48.2,21.9 48.4,22.1 | v13,14.3 13,15 12.8,15.2 11.2,15.2 9.6,13.6 R23.2
  Top 0.203: U6.5 48.4,22.1
  Top 0.254: R22.2 12.6,13.3 13,13.7 v13,14.3
  Bottom 0.2: v48.2,21.6 48.2,15.9 47.2,14.9 43.2,14.9 39.2,10.9 13.9,10.9 13,11.8 v13,14.3
N$40  (via drill 0.6)
  other vias: 2.9,12.4
N$41
  Top 0.2: B0.B B0.B1 42.3,10.3 42,10.6 41.15,10.6 R61.1
N$42
  Top 0.203: R15.2 89.35,47.55 92.3,50.5
  Top 1: RCA-VIDEO-OUT.2 94.6,52.1 93.9,52.1 92.3,50.5
N$43
  Top 0.406: C53.1 3.3,44.2 3.65,43.85 R51.2 C55.1
N$44
  Top 0.406: TV6.1 5.05,46.85 5,46.9 5,48.4 4,49.4 CN7.4 | R40.1 5.1,45.2 5.05,45.25 TV6.1 | C53.2 3.3,46.9 3.4,46.8 TV6.1
N$45
  Top 0.406: R49.1 10.2,45.2 10.15,45.25 10.15,46.54 | 10.15,46.54 TV5.1 10.15,47.05 10.2,47.1 10.2,47.7 9.2,48.7 CN7.1 | 10.15,46.54 10.24,46.54 10.5,46.8 11.9,46.8 C54.2
N$46  (via drill 0.5)
  Top 0.25: U7.8 U7.7 35.2,49.9 v35.6,50.3 | R38.1 15.85,42.25 Q1.C
  Top 0.305: 15.85,42.25 15.85,47.55 v16.6,48.3
  Top 0.406: 15.9,38.1 R38.1 R39.2
  Bottom 0.305: v35.6,50.3 25.8,50.3 24.7,51.4 19.7,51.4 v16.6,48.3
N$47
  Top 0.203: U30.2 63.3,45.55 C46.2
N$48
  Top 0.203: U30.3 62.65,44.85 62.3,45.2 61.7,45.2 61.1,45.7 61.1,45.75 C58.2
N$51
  Top 0.203: U30.15 63.3,36.5 63.8,36 65.35,36 JMP5.2
N$52
  Top 0.305: TV1.1 93.4,46.1 | R15.1 TV1.1 | TV1.1 92.3,46.1 92.1,45.9 92,45.9 | 92,45.9 91.9,46 | 92,45.9 92.1,45.8 92.1,45.7 | R10.2 92.05,44.25 92.1,44.3 92.1,45.7 | 92.1,45.7 92.4,46 | 92.1,45.7 91.8,46
N$57
  Top 0.2: R54.2 LED2.A
N$58
  Top 0.2: R55.2 39.15,14.6 LED1.A
N$59
  Top 0.25: U7.1 36.7,45.6 37.6,44.7 38.5,44.7 39.1,44.1 J2.2
N$60
  Top 0.2: R56.2 34.45,14.6 LED3.A
N$61
  Top 0.25: U7.15 32.7,45.6 31.8,44.7 30.7,44.7 30.15,44.15 J1.2
N$62
  Top 0.25: U7.2 39.3,46.7 40.4,47.8 40.4,49.6 39.5,50.5 39.2,50.5 L4.1
N$63
  Top 0.25: U7.5 36.7,48.3 36.6,48.4 36.6,50.4 37.1,50.9 L5.1
N$64
  Top 0.2: R19.1 44.6,55.8 44.23,56.17 JP2.2
N$65
  Top 0.406: L5.2 37.1,55.4 37,55.5 37.05,55.55 C43.1 37.05,56.65 36.7,57 36.7,58.2 36.5,58.4 JPL.2
N$66
  Top 0.25: L3.1 32.2,50.9 32.7,50.4 U7.11
N$67
  Top 0.406: L3.2 32.2,54.7 32.3,54.8 32.3,55.6 C41.1 32.35,56.65 32.7,57 32.7,58.1 33,58.4 JPR.2
N$68
  Top 0.25: U7.14 30,46.7 28.8,47.9 28.8,49.4 29.9,50.5 30.2,50.5 30.6,50.9 L2.1
N$69
  Top 0.254: R20.2 25.65,35.75 25.6,35.7 25.6,33.5 26.66,32.44 U8.7 27.64,32.44 | R21.1 30.45,34.35 28.7,32.6 28.6,32.6 28.5,32.5 27.7,32.5 27.64,32.44 | 27.64,32.44 27.6,32.4
N$70
  Top 0.2: R1.2 50.45,44.95 50.4,44.9 50.75,44.55 C13.2 | 49.6,42.1 50.2,42.7 50.4,42.7 XT1.3
  Top 0.203: U6.44 49.6,42.1
  Top 0.3: XT1.3 50.6,43 50.45,43.15 R1.2
N$71
  Top 0.2: XT1.1 48.6,41.4 49.2,40.8
  Top 0.203: U6.45 49.2,40.8
  Top 0.3: XT1.1 48.4,41.3 48.3,41.4 47.3,41.4 46,42.7 46,43.4 47.1,44.5 C12.2 48.35,44.55 48.75,44.95 R1.1
N$72
  Top 0.203: U30.8 59.4,41.4 59.1,41.1 C63.1
N$73
  Top 0.203: U30.7 60.05,42.05 61.1,41 64.6,41 65.3,40.3 67.5,40.3 68.5,41.2 69.25,41.2 JMP4.2
N$88
  Top 0.254: U8.3 21.35,31.15 21.3,31.1 21.3,30.6
  Top 0.305: U8.3 21.62,31.18 21.7,31.1 21.7,30.1 21.5,29.91 U8.4
  Top 0.406: 17.6,30.57 17.6,30.6
  Top 1: 17.6,30.6 R63.1
  Top 1.016: 21.3,30.6 19.4,30.6 19.25,30.45 C52.1 19.2,30.5 19.1,30.6 17.6,30.6
N$89
  Top 0.2: B2.B B2.B1 25.5,12.1 25.3,12.3 24.45,12.3 R37.1
N$90
  Top 0.2: SW2.2 91.8,38.8 92.1,38.5 94,38.5 94.4,38.9 94.4,42.3 93.8,42.9 93.8,44.15 R10.1
N$95
  Top 0.2: JP4.1 89.97,41.37 SW2.3 91.14,40.2 92.4,40.2 93.15,39.45 R26.1
N$96
  Top 0.2: JP4.2 87.17,38.83 88.5,37.5 91.5,37.5 92.8,36.2 92.95,36.2 R25.1
N$100
  Top 0.2: B3.B B3.B1 17.1,8.9 17.9,9.7 17.9,11.5 17.3,12.1 17.15,12.1 R36.1 C20.2
R+
  Top 0.406: L2.2 30.6,54.5 30.9,54.8 30.9,55.6 C40.1 31.05,56.55 30.7,56.9 30.7,58.1 30.43,58.37 JPR.1
RIGHT  (via drill 0.5)
  Top 0.2: JP6.1 34.8,34.5
  Top 0.23: U6.60 43.5,29.2
  Top 0.25: 43.5,29.2 41.1,31.6 38,31.6 35.12,34.48 JP6.1
  Top 0.406: R5.1 22.25,43.15 22.2,43.1 | R5.1 R17.1 | R13.2 32.7,39.6 33.6,38.7 v33.6,38.6 | R5.1 22.3,43.3 | v21.1,43.3 R5.1 | R50.1 13.25,43.55 13.5,43.8 v13.5,44.8
  Bottom 0.406: JP6.1 34.8,37.4 33.7,38.5 | 33.7,38.5 v33.6,38.6 | 33.7,38.5 25.9,38.5 v21.1,43.3 15,43.3 v13.5,44.8
RTCVDD  (via drill 0.4, 0.5)
  Top 0.203: D6.CATHODE 33.7,20.2 v33.3,19.8
  Top 0.23: U6.55 44.8,31.2
  Top 0.25: 44.8,31.2 43.79,32.29 v43.8,33.3
  Top 0.3: v33.3,19.8 33.75,19.8
  PWR 0.305: v43.8,33.3 43.79,29.17 46.7,26.2 46.7,23.7 45.4,22.4 44.9,22.4 43.4,23.9 43.4,24.3 42.8,24.9 38.3,24.9 35.1,21.7 29.7,21.7 29,21 29,20.3 29.5,19.8 v33.3,19.8 40.6,19.8 41.1,19.3 41.1,11.7 46.8,6 BATT2.P2
  Bottom 0.2: BATT2.P1 59.9,4 59.5,3.6 47.1,3.6 46.7,4 BATT2.P2 46.7,6.1
RX0  (via drill 0.5)
  Top 0.2: 58.1,29.6 58.8,28.9 58.8,26.1 v58.9,26
  Top 0.203: U6.27 58.1,29.6
  Top 0.61: JP1.16 81.57,40.77 81.6,40.8 81.65,40.75 R34.1
  Bottom 0.2: v58.9,26 58.8,26.1 58.8,28.9 58.1,29.6 56.5,29.6 53.8,32.3 53.8,34.4 54.5,35.1 55.6,35.1 57.2,33.5 63,33.5 64.2,34.7 67,34.7 67.4,34.3 73.5,34.3 78.7,39.5 80.3,39.5 81.57,40.77 | 81.57,40.77 81.6,40.8 | 81.57,40.77 JP1.16
RX1  (via drill 0.5)
  Top 0.2: 47.6,34 45.6,36 45.6,38 46.2,38.6 v46.2,39 | R35.1 76.9,53.4 77,53.5 79.1,53.5 79.05,53.45 JP1.5
  Top 0.203: U6.49 47.6,34
  Bottom 0.2: v46.2,39 46.2,39.1 51.1,44 53.5,44 54.5,43.1 54.5,42.6 56.1,41 62.6,41 63.6,42 67.6,42 79.03,53.43 JP1.5 79.05,53.45 80.2,54.6 87.5,54.6 95.7,46.4 95.7,42.88 JP15.1
SCK0  (via drill 0.4, 0.5, 0.6)
  Top 0.2: U2.30 72.05,25.45 v67.4,20.8 66.2,19.6 66.2,16.1 65.1,15 v64.4,15 | v64.4,15 62.4,15 62.37,14.96 U4.6 | 64.36,14.96 v64.4,15 | v54.65,38.25 54.6,38.2 54.6,37.4 51.6,34.4 | v14.9,2.9 B3.A B3.A1 13.1,8.9 14.1,9.9 R62.1 C20.1
  Top 0.203: U6.39 51.6,34.4
  GND 0.2: v75.8,20.4 75,21.2 67.8,21.2 v67.4,20.8
  Bottom 0.152: U$37.B2 78,19.6 77,19.6 76.2,20.4 v75.8,20.4
  Bottom 0.2: v64.4,15 63,16.4 61.4,16.4 60.1,17.7 60.1,22.6 58.3,24.4 55.9,24.4 | 54.5,38.2 54.55,38.25 v54.65,38.25 54.3,37.9 53.1,37.9 51,35.8 | v14.9,2.9 16.1,1.7 62.3,1.7 62.9,2.3 62.9,7.6 66.7,11.4 | 66.7,11.4 66.8,11.5 66.8,12.5 67.5,13.2 67.5,20.7 v67.4,20.8 | JP5.4 69.96,8.14 66.7,11.4
  Bottom 0.203: 55.9,24.4 55.8,24.4 52.9,27.3 48.8,27.3 48.2,27.9 48.2,30.5 48.7,31 50.3,31 50.9,31.6 50.9,35.7 51,35.8
SCK1  (via drill 0.5)
  Top 0.2: v56.08,28.45 56.08,28.48 56.1,28.5 55.8,28.8 | R27.2 68.45,35.55 v67.9,36.2
  Top 0.203: U6.25 55.8,28.8
  Bottom 0.2: v56.08,28.45 56.08,28.82 53,31.9 53,34.8 54.1,35.9 58,35.9 59.1,37 65.8,37 66.7,36.1 67.6,36.1 v67.9,36.2 68.5,36.3 71,36.3 71.8,35.5 72.8,35.5 77.6,40.3 77.6,41.1 78.6,42.1 80.4,42.1 81.59,43.29 | 81.59,43.29 81.6,43.3 | 81.59,43.29 JP1.14
SCK1_  (via drill 0.5)
  Top 0.2: U2.46 70.15,30.75 69.6,31.3 69,31.3 | 69,31.3 68.6,31.7 68.6,32.5 69.2,33.1 R27.1 | 69,31.3 v68.8,31.1
  Bottom 0.152: U$37.D5 80.7,13.8 80.5,13.6
  Bottom 0.2: 80.5,13.6 73.2,13.6 72.9,13.9 72.9,18.3 72.5,18.7 72.5,26.4 72.8,26.7 72.8,27.6 72.55,27.85 72.55,28.95 70.4,31.1 v68.8,31.1
SDTO
  Top 0.2: U30.9 59.4,34.84 JP16.P$2
SPDIFI  (via drill 0.5)
  Top 0.2: 50,23.2 51.9,21.3 53.1,21.3 54,20.4 v54,19.7
  Top 0.203: U6.9 50,23.2
  Bottom 0.2: v54,19.7 54,21 | 50.2,36.2 50.7,36.7 50.7,38.3 51.4,39 53.7,39 54.1,39.4 63.4,39.4 64.4,40.4 69.9,40.4 71.1,41.6 72.26,41.6 JP1.9 79,48.4
  Bottom 0.203: 50.2,36.2 50.1,36.1 50.1,33.6 47.4,30.9 47.4,27.5 48.4,26.5 50.1,26.5 54,22.6 54,21
SPDIFO  (via drill 0.5)
  Top 0.2: 50.4,23.4 52.1,21.7 53.6,21.7 55.9,19.4 v56,19.4
  Top 0.203: U6.10 50.4,23.4
  Bottom 0.2: v56,19.4 56,17.6 55,16.6 53.2,16.6 52.2,17.6 52.2,19.8 | 49.8,36.4 50.3,36.9 50.3,38.5 51.2,39.4 53.5,39.4 53.9,39.8 63.2,39.8 64.2,40.8 69.7,40.8 78.5,49.6 80.3,49.6 81.6,50.9 81.59,50.91 JP1.8
  Bottom 0.203: 49.8,36.4 49.7,36.3 49.7,33.8 47,31.1 47,27.3 52.2,22.1 52.2,19.8
SPK0  (via drill 0.5, 0.6)
  Top 0.2: 46.4,33.2 46.1,33.5 46.1,34.2 44.7,35.6 44.7,37 44,37.7 44,39.5 45.3,40.8 v45.3,40.9 | R19.2 46.35,55.65 45,54.3 45,54.2 44.6,53.8 | 44.6,53.8 R18.1 | v43.3,53.8 44.6,53.8
  Top 0.203: U6.51 46.4,33.2
  Top 0.3: v45.3,40.9 45.3,44.1 v45.1,44.3
  Bottom 0.2: v45.3,40.9 46.6,40.9 50.6,44.8 55.2,44.8 58.2,41.8 61.9,41.8 64.4,44.3 66,44.3 67.7,46 67.7,47.6 76.1,56 JP1.3
  Bottom 0.254: v45.3,40.9 45.3,40.8 | 43,48.1 43,53.5 v43.3,53.8
  Bottom 0.3: v45.1,44.3 45.1,45.9 43,48 43,48.1
SPK1  (via drill 0.5)
  Top 0.2: 46,32.8 45.7,33.1 45.7,34 44.3,35.4 44.3,36.8 43.6,37.5 43.6,40.4 v44.1,40.9 | v64,47.1 64,46 64.2,45.8 64.2,44.6 64.4,44.4 70.8,44.4 71.9,43.3 71.9,41.8 76.7,37 85.3,37 88.4,33.9 89.1,33.9 90.4,32.6 CN3.11 | R12.1 27.35,27.15 v27.4,27.2
  Top 0.23: 46,32.8 U6.52
  Top 0.61: R12.1 27.35,25.55 27.1,25.3 U5.1
  PWR 0.2: v27.4,27.2 28.1,26.5 32,26.5 33.6,28.1 35.5,28.1 36.7,29.3 36.7,33.5 v44.1,40.9
  Bottom 0.2: v64,47.1 64,45.5 60.7,42.2 58.4,42.2 55.4,45.2 50.3,45.2 47,41.9 45.2,41.9 v44.1,40.9
TX0  (via drill 0.5)
  Top 0.2: 58.3,30 59.2,29.1 59.2,26.8 v60.05,25.95
  Top 0.203: U6.28 58.3,30
  Bottom 0.2: v60.05,25.95 59.2,26.8 59.2,29.1 58.3,30 56.7,30 54.2,32.5 54.2,34.2 54.7,34.7 55.4,34.7 57,33.1 63.2,33.1 64.4,34.3 66.8,34.3 67.2,33.9 74.7,33.9 79.01,38.21 JP1.17
TX1  (via drill 0.5)
  Top 0.2: 48,34.2 46.4,35.8 v46.4,36.6
  Top 0.203: U6.48 48,34.2
  Bottom 0.2: v46.4,36.6 48.2,36.6 49.1,37.5 49.1,40.8 51.9,43.6 53.3,43.6 54.1,42.8 54.1,42.4 55.9,40.6 62.8,40.6 63.8,41.6 68,41.6 78.6,52.2 80.4,52.2 81.6,53.4 | 81.6,53.4 81.57,53.43 JP1.6 | 81.6,53.4 82,53.4 83.6,51.8 83.6,47.7 86.5,44.8 91.6,44.8 94.8,41.6 98.7,41.6 99.3,41 99.3,36.32 JP15.8
USB1_N
  Top 0.192: 44.27,26.8 42.18,24.71 38.58,24.71 35.6,21.8 33,21.8 32.5,21.3 32.5,18.63 30.68,16.81 | SW1.5 13.7,19.5 14.7,18.5 16,18.5 16.31,18.19 16.31,17.62 17.12,16.81 21.5,16.81 21.96,16.35 R32.2 22.35,16.6 22.5,16.6 22.71,16.81
  Top 0.2: 30.68,16.81 28.74,16.81 arc-90 28.03,17.52 arc90 27.7,17.85 27.44,17.85 arc90 27.11,17.52 arc-90 26.4,16.81 22.71,16.81 | U6.66 44.27,26.8
USB1_P
  Top 0.192: 44.13,27.2 42.02,25.09 38.42,25.09 35.5,22.2 32.6,22.2 32.1,21.7 32.1,18.77 30.52,17.19 | 22.71,17.19 22.5,17.4 22.35,17.4 R33.2 21.96,17.65 21.5,17.19 21.4,17.19 arc-90 21.06,17.53 21.06,17.68 arc90 20.73,18.02 20.67,18.02 arc90 20.34,17.68 20.34,17.53 arc-90 20,17.19 19.94,17.19 arc-90 19.61,17.53 19.61,17.68 arc90 19.27,18.02 19.21,18.02 arc90 18.88,17.68 18.88,17.53 arc-90 18.54,17.19 17.28,17.19 16.69,17.78 16.69,19.21 16.4,19.5 SW1.2
  Top 0.2: 30.52,17.19 28.74,17.19 arc-90 28.41,17.52 arc90 27.7,18.24 27.44,18.24 arc90 26.73,17.52 arc-90 26.4,17.19 22.71,17.19 | U6.65 44.13,27.2
USB2_N
  Top 0.192: SW1.6 12.85,22.3 | 12.74,22.65 6.05,29.34 6.05,31.95
  Top 0.2: 12.85,22.3 12.85,22.54 12.74,22.65
  Top 0.25: 6.05,31.95 8.19,34.09 X2.2
USB2_P
  Top 0.192: 14.16,22.65 13.26,22.65 6.45,29.46 6.45,31.8 6.85,32.2 X2.3
  Top 0.2: 14.16,22.65 15.31,21.5 SW1.3
USB3_N
  Top 0.192: X1.2 6.99,18.3 7.2,18.09 7.86,18.09 arc90 8.2,18.43 8.2,18.84 arc-90 8.53,19.17 8.55,19.17 arc-90 8.88,18.84 8.88,18.43 arc90 9.22,18.09 9.24,18.09 arc90 9.57,18.43 9.57,18.84 arc-90 9.91,19.17 9.93,19.17 arc-90 10.26,18.84 10.26,18.43 arc90 10.6,18.09 11.38,18.09 11.94,17.54 12.81,17.54 SW1.4
USB3_P
  Top 0.192: X1.3 6.99,17.5 7.2,17.71 11.22,17.71 11.66,17.26 11.67,17.26 12.43,16.5 14.35,16.5 SW1.1
USBVDD
  Top 0.2: 44,26 43.3,25.3 43.3,24.7 42.2,23.6 JP9.1
  Top 0.23: U6.68 44,26
  Top 0.61: C14.1 42.06,23.36 JP9.1
VD4  (via drill 0.5)
  Top 0.2: U2.20 72.65,22.15 72.8,22.3 75.1,22.3 77,20.4 78.5,20.4 v79.3,21.2 83.9,21.2 84.4,20.7 85.1,20.7 86.9,18.9 96.1,18.9 97.4,20.2 97.4,31.7 99.3,33.6 99.3,41.2 98.9,41.6 96.96,41.6 JP15.3
  Bottom 0.152: U$37.C1 79.7,20.8 v79.3,21.2
VD5  (via drill 0.5)
  Top 0.2: U2.19 72.15,22.45 72.4,22.7 75.3,22.7 76,22 80,22 80.4,21.6 v84.9,21.6 87.2,19.3 95.9,19.3 97,20.4 97,39.1 JP15.4
  Bottom 0.2: U$37.E5 83.6,15.9 83.9,16.2 83.9,20.6 v84.9,21.6
VD6  (via drill 0.5)
  Top 0.2: U2.41 72.65,29.25 72.8,29.1 74.4,29.1 74.6,28.9 v74.6,28.3
  Bottom 0.152: U$37.E3 81.2,18.4 81.2,19.2 81,19.4 80.4,19.4 80.2,19.6 80.2,21.5 79.2,22.5 78.2,22.5 77.1,23.6 77.1,25.8 v74.6,28.3
  Bottom 0.2: v74.6,28.3 74.6,31.7 75.6,32.7 91,32.7 91,32.8 94.7,36.5 96.94,36.5 JP15.6
VDOUT0  (via drill 0.5)
  Top 0.2: U2.7 70.85,25.45 71.8,26.4 72.8,26.4 73.3,26.9 v73.3,28.3
  Bottom 0.152: U$37.C5 79.7,14.2 79.5,14
  Bottom 0.2: SW2.1 90,35.1 88,33.1 75.4,33.1 73.3,31 v73.3,28.3 73.3,26.6 72.9,26.2 72.9,18.9 73.3,18.5 73.3,14.1 73.4,14 79.5,14
VHIGH  (via drill 0.5, 0.6)
  Top 0.2: PWR.B PWR.B1 8.5,8.5 | C44.2 11.1,13.8 v11.6,14.3 | 8.5,8.5 8.4,8.5 | v7.1,9.8 7.9,9.8 8.3,9.4 8.3,8.7 8.5,8.5
  Top 0.406: X1.1 6.01,20.18 v6.5,20.2 v5.2,20.2 | v5.2,20.2 v7.8,20.2 7.1,19.4 6.9,19.2 | 5.1,19.2 5.1,20.1 v5.2,20.2
  Top 0.61: U5.4 24.1,20.7 24.05,20.75 C36.1 20.75,20.75 v20.7,20.7 v19.5,20.7
  PWR 0.2: 20.9,19 20.9,19.5 20.7,19.7 | 20.7,19.5 21.3,18.9
  PWR 0.254: 20.6,18.8 20.8,18.8 21,19 20.9,19
  PWR 0.406: 26.4,37.7 26.4,44.3 26.4,51.4 30.5,55.5 39.2,55.5 40.2,56.5 52.1,56.5 53.1,55.5 55.3,55.5 55.8,56 56.7,56 57.2,55.5 64.5,55.5 67.5,58.5 79.1,58.5 79.07,58.53 JP1.1
  PWR 0.61: v19.5,20.7 19.5,19.6 19.6,19.5 19.8,19.5 20,19.3 20.5,19.3 20.7,19.5 20.7,19.7 20.7,20.6 20.1,20.6 20.1,18.62 20.1,18.6 | 1.9,9 1.9,4.8 2.7,4 26.3,4 28.3,6 40.9,6 44.9,2 86.6,2 87.2,2.6 87.2,8.5 87.3,8.6 87.2,8.7 CN2.5
  PWR 1.016: 12.8,30.4 12.9,30.3 12.8,30.2 12.8,27.5 17.6,22.7 17.6,20.6 19.58,18.62 | X2.1 10.6,34.3 10.6,32.6 12.8,30.4 | 12.8,30.4 JP3.2 | 19.58,18.62 20.1,18.62 | 19.6,18.6 19.58,18.62 | 20.9,18.6 20.8,18.6 20.6,18.8
  pour PWR (isolate 0.305, rank 2): 0.1,8.9 0.1,38 42.1,38 42.1,8.9
VXTALI
  Top 0.2: U2.32 77.55,26.45 79.7,24.3 JP14.3 83.11,24.16 C34.2 | C34.2 83.5,24.5 83.29,24.29 | C34.2 R57.2
  Bottom 0.152: U$37.D1 80.7,21.6 79.7,22.6 JP14.3
VXTALO
  Top 0.2: U2.33 77.55,26.95 79.7,29.1 JP14.1 83.11,29.24 C35.2 | C35.2 83.5,28.8 83.19,29.11 | 83.5,27.5 R57.1 C35.2
  Bottom 0.152: U$37.E1 81.7,21.7 82.1,22.1 82.1,28.7 81.5,29.3 79.76,29.3 JP14.1
XCS  (via drill 0.5)
  Top 0.2: 54.6,26.4 54.7,26.3 54.7,25.4 55.3,24.8 v60.5,24.8 | U2.48 67.55,29.95 v67.2,30.3 67.2,31.5 67.3,31.6 67.3,31.65 R58.2
  Top 0.203: U6.19 54.6,26.4
  GND 0.2: v76.3,19.3 76.9,19.9 76.9,20.8 75.8,21.9 68.5,21.9 67.6,22.8 67.6,29.9 v67.2,30.3
  Bottom 0.152: U$37.C2 79.2,18.4 77.2,18.4 v76.3,19.3
  Bottom 0.2: v60.5,24.8 60.77,25.07 63,25.07 63.4,25.47 63.4,29.8 63.9,30.3 65,30.3 65.6,30.9 66.6,30.9 v67.2,30.3
XCS0  (via drill 0.4, 0.5)
  Top 0.2: 49.2,22.8 51.5,20.5 52.5,20.5 52.6,20.4 52.6,19.4 54.3,17.7 | 54.3,17.7 54.5,17.5 U4.1 | 54.3,17.7 v54,17.4 53.8,17.4 52.9,16.5 48.4,16.5 47.2,15.3 44.9,15.3 44.3,15.9 42.3,15.9 41.8,15.4 41.8,14.45 R2.2 43.12,13.17 JP7.2
  Top 0.203: U6.7 49.2,22.8
  PWR 0.2: v60.4,8.6 63.75,8.6 JP5.1
  Bottom 0.2: v54,17.4 54,18.5 54.8,19.3 | 50.6,36 51.1,36.5 51.1,38.1 51.6,38.6 53.9,38.6 54.3,39 63.6,39 64.6,40 70.1,40 71.1,41 72.4,41 78.5,47.1 80.3,47.1 JP1.10 81.6,48.4 | JP7.2 46.63,13.17 48.3,11.5 48.3,10.3 50,8.6 v60.4,8.6
  Bottom 0.203: 50.6,36 50.5,35.9 50.5,31.9 50,31.4 48.5,31.4 47.8,30.7 47.8,27.7 48.6,26.9 50.4,26.9 54.8,22.5 54.8,19.3
XCS1  (via drill 0.5)
  Top 0.2: 57.7,29.2 58,28.9 v58,26.8 | R25.2 93.35,37.55 94.4,36.5 94.4,35.2 93.9,34.7 88.5,34.7 85.7,37.5 84.2,37.5 82.2,39.5 80.28,39.5 JP1.15
  Top 0.203: U6.26 57.7,29.2
  Bottom 0.2: v58,26.8 58,28.9 57.7,29.2 56.3,29.2 53.4,32.1 53.4,34.6 54.3,35.5 58.2,35.5 59.2,36.5 65.5,36.5 66.7,35.3 67,35.3 67.6,34.7 73,34.7 79.05,40.75 | 79.05,40.75 79.1,40.8 | 79.05,40.75 JP1.15
XHLD0  (via drill 0.4, 0.5, 0.6)
  Top 0.2: U2.31 71.95,25.95 67.9,21.9 66.6,21.9 65.8,21.1 65.8,17.7 v65.4,17.7 | v52.7,40.9 52.7,37.3 50.4,35 | v40.2,2.8 38.4,2.8 B0.A B0.A1 38.3,12.1 38.1,12.3 37.25,12.3 R30.1 | v65.6,11.9 67.2,11.9 69.8,9.3 71.2,9.3 72.5,8 JP5.6
  Top 0.203: U6.42 50.4,35
  GND 0.2: v65.4,17.7 69.1,14 81.4,14 v81.7,14.3
  Bottom 0.152: U$37.D4 80.8,16.9 81.2,16.5 81.2,14.8 v81.7,14.3
  Bottom 0.2: 51.8,20 51.8,15.9 49,13.1 49,10.6 50.4,9.2 60.7,9.2 62.1,7.8 | v65.4,17.7 66.9,16.2 66.9,13.3 66.4,12.8 66.4,12.7 v65.6,11.9 65.6,10.9 62.5,7.8 | 49.4,36.6 49.55,36.75 49.9,37.1 49.9,40.4 50.4,40.9 v52.7,40.9 | 62.3,7.6 62.5,7.8 | 62.3,7.6 62.3,4.5 60.6,2.8 v40.2,2.8 | 62.3,7.6 62.1,7.8 | 62.5,7.8 62.1,7.8
  Bottom 0.203: 49.55,36.75 49.3,36.5 49.3,34 46.6,31.3 46.6,27 51.8,21.8 51.8,20
XHLD1  (via drill 0.5, 0.6)
  Top 0.2: 47.2,33.8 45.2,35.8 45.2,38 44.8,38.4 v44.8,39 | R56.1 v31.4,16.1
  Top 0.203: U6.50 47.2,33.8
  Bottom 0.2: 81.4,56 80.7,56 79.4,54.7 75.4,54.7 68.1,47.4 68.1,45.8 66.1,43.7 64.5,43.7 62.1,41.4 56.2,41.4 54.9,42.7 54.9,43.2 53.7,44.4 50.8,44.4 46.4,40 45.8,40 v44.8,39 44.8,35.9 | 46.3,17.1 45,15.8 38.1,15.8 36.9,17 32.3,17 v31.4,16.1
  Bottom 0.203: 44.8,35.9 44.8,35 45.7,34.1 45.7,26.5 46.9,25.3 46.9,17.7 46.3,17.1
  Bottom 0.25: JP1.4 81.41,55.99 81.4,56
XSHDN  (via drill 0.5)
  Top 0.2: v49.3,21.6 49.3,21.8 48.8,22.3 | v11.2,38.1 R39.1
  Top 0.203: U6.6 48.8,22.3
  Bottom 0.2: v49.3,21.6 49.3,16 47.8,14.5 43.9,14.5 39.5,10.1 11.7,10.1 10.7,11.1 10.7,37.6 v11.2,38.1
XWP0  (via drill 0.4, 0.5, 0.6)
  Top 0.2: 50.8,23.6 52.3,22.1 53.8,22.1 55.6,20.3 56.3,20.3 57.2,19.4 v57.2,19.2 | U2.10 66.95,23.95 65.4,22.4 v59.2,22.4 | v52.8,14.2 52.4,14.6 50.7,14.6 49,12.9 49,9.6 47.8,8.4 45.4,8.4 44.4,7.4 44.4,1.8 44.1,1.5 30.1,1.5 29.9,1.7 B1.A B1.A1 29.9,12.2 29.7,12.4 28.95,12.4 R31.1 | v78.9,14.8 v78.9,11.3
  Top 0.203: U6.11 50.8,23.6
  GND 0.2: v78.9,14.8 69.5,14.8 65.6,18.7 63.8,18.7 63.3,19.2 63.3,21.6 62.5,22.4 v59.2,22.4
  Bottom 0.152: U$37.C4 79.2,16.4 79.2,15.1 v78.9,14.8
  Bottom 0.2: v59.2,22.4 57.3,20.5 57.3,19.2 v57.2,19.2 57.2,15.9 55.5,14.2 v52.8,14.2 | v78.9,11.3 79.6,10.6 79.6,3.7 78.7,2.8 73.2,2.8 72.5,3.5 JP5.5
XWP1  (via drill 0.5, 0.6)
  Top 0.2: v48,35.7 48.4,35.2 | R55.1 v36,16.1
  Top 0.203: U6.47 48.4,35.2
  Bottom 0.2: 79.01,50.91 69.3,41.2 64,41.2 63,40.2 55.8,40.2 54,42 50.9,42 49.5,40.6 49.5,37.3 48,35.8 v48,35.7 48,34.6 47.3,33.9 | 47.3,15.7 46.9,15.3 36.8,15.3 v36,16.1
  Bottom 0.203: 47.3,33.9 46.2,32.8 46.2,26.7 47.4,25.5 47.4,15.8 47.3,15.7
  Bottom 0.25: JP1.7 79.01,50.91

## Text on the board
Top: 1
GND: 2
PWR: 3
Bottom: VS1010 Developer Board | V2.0 | PL/HV 2019 | 4
tPlace: IOVDD | ADC / in | VHIGH | XHLD1 | LIN | TX1 | HP | LOUT | SPK0 | RX1 | SPDIFO | XWP1 | XCS0 | SPDIFI | CVDD | MOSI1 | SCK1 | MISO1 | XCS1 | RX0 | TX0 | i2s data | ADC | AVDD | R | I2S | 12M | BCK | GND | GBUF | DI | FRM | DO | ioV | ANA / PWR | L | AVDD | GND | 1 | GND | GND | VS1010 / DevBoard / v.2.0 | GND CS0 | IOVDD | SCK0 | XHLD0 | GND | Mouse / DATA | MISO0 | XWP0 | MOSI0 | Mouse / CLK | XCS0
bPlace: RX1 | VD5 | G | VD4 | VS1010 Developer Board | GP2_7 | V2.0 | 3V3 | TX1 | VD6 | T.H 2017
